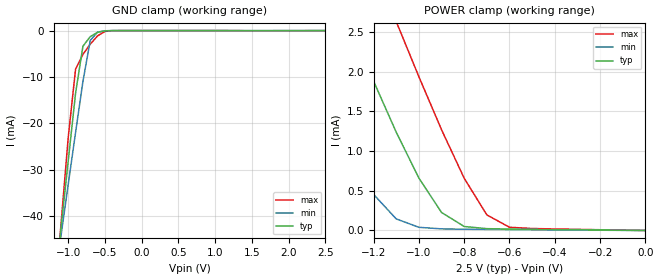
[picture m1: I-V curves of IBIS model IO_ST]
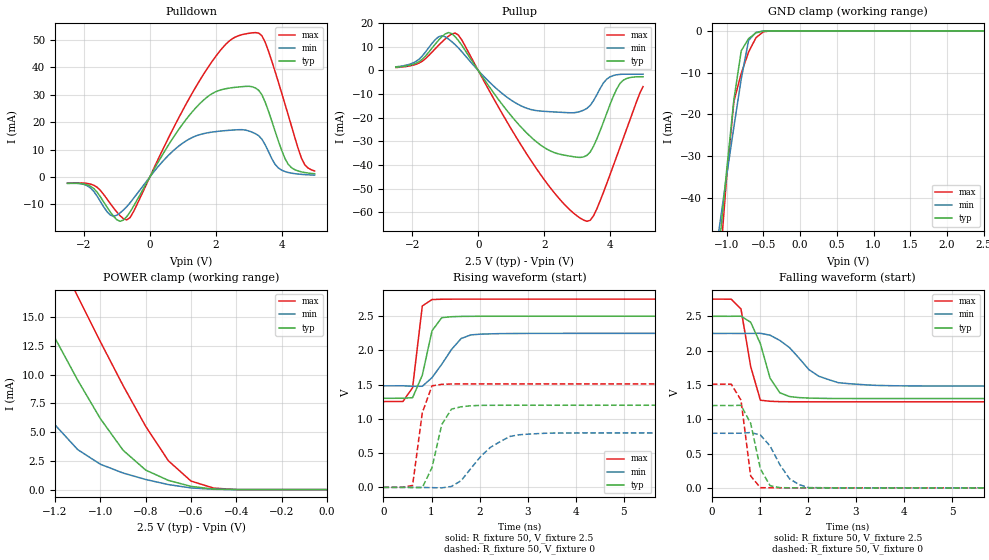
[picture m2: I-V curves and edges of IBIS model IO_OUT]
[IBIS Ver]   3.2
[Comment Char]   |_char
[File name]   sg5032can25.ibs
[File Rev]   1.0
[Date]   2015/11/24 22:00:00
[Source]
[Notes]
[Disclaimer]
This information is for modeling purposes only, and is not guaranteed.
Property of SEIKO EPSON Corp.,
unauthorized reproduction and/or distribution is strictly prohibited.
[Copyright]
Copyright 2006, SEIKO EPSON Corp.
[Component]   SG5032CAN
Si_location Pin
Timing_location Pin
[Manufacturer]   SEIKO EPSON Corp.
| COG
| COG
[Package]
R_pkg   56.75m   56.75m   56.75m
L_pkg   2.25n   2.25n   2.25n
C_pkg   0.860p   0.860p   0.860p
[Pin] signal_name   model_name
1   /ST   IO_ST
2   GND   GND
3   OUT   IO_OUT
4   Vcc   POWER
| Models and submodels in the file (2): IO_ST (Input), IO_OUT (3-state)
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[Model]   IO_ST
Model_type Input
Polarity Inverting
Vinh=2.00
Vinl=0.50
C_comp   5p   4p   6p
[Temperature Range] 25   105   -40
[Voltage Range]   2.5   2.25   2.75
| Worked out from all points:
|   GND clamp passes 1 mA (typ) near -0.67 V on its own axis
|   POWER clamp passes 1 mA (typ) near -1.06 V on its own axis
[GND Clamp]
-2.5V     -258mA     -212mA     -315.4mA
-1.2V     -57.55mA   -55.73mA   -61.1mA
-1.1V     -42.76mA   -44.37mA   -42.03mA
-1V       -28.06mA   -33.1mA    -23.01mA
-900mV    -13.48mA   -21.96mA   -8.306mA
-800mV    -3.366mA   -10.96mA   -5.116mA
-700mV    -1.291mA   -2.106mA   -2.915mA
-600mV    -372.4uA   -316.5uA   -1.133mA
-500mV    -49.9uA    -42.12uA   -183.6uA
-400mV    -3.838uA   -5.008uA   -10.26uA
2.5V      36.41pA    4.239uA    -10.27uA
[POWER Clamp]
-2.5V     10.82mA    8.867mA    12.49mA
-1.6V     4.625mA    2.831mA    6.156mA
-1.5V     3.936mA    2.166mA    5.451mA
-1.3V     2.559mA    943.7uA    4.043mA
-1.2V     1.882mA    455uA      3.338mA
-1.1V     1.239mA    146uA      2.634mA
-1V       661uA      40.15uA    1.938mA
-900mV    227.3uA    20.05uA    1.27mA
-800mV    50.18uA    15.52uA    658.6uA
-700mV    22.76uA    13.11uA    196.3uA
-600mV    17.66uA    11.02uA    40.37uA
0V        36.41pA    613.4pA    26.22pA
[Model]   IO_OUT
Model_type 3-state
Enable Active-High
Polarity Non-Inverting
Vmeas=1.25
C_comp   5p   4p   6p
[Temperature Range] 25   105   -40
[Voltage Range]   2.5   2.25   2.75
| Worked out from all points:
|   slope of the pulldown table from 0 to 0.375 V, typ, clamps not added: 47.4 ohm
|   slope of the pullup table from 0 to 0.375 V, typ, clamps not added: 48.9 ohm
|   GND clamp passes 1 mA (typ) near -0.64 V on its own axis
|   POWER clamp passes 1 mA (typ) near -0.72 V on its own axis
|   falling waveform, R_fixture 50, V_fixture 2.5: 20-80 % time 358ps typ, 689ps min, 253ps max; typ from 2.5 V to 1.3 V
|   falling waveform, R_fixture 50, V_fixture 0: 20-80 % time 246ps typ, 411ps min, 166ps max; typ from 1.2 V to 0 V
|   rising waveform, R_fixture 50, V_fixture 2.5: 20-80 % time 253ps typ, 473ps min, 152ps max; typ from 1.3 V to 2.5 V
|   rising waveform, R_fixture 50, V_fixture 0: 20-80 % time 274ps typ, 666ps min, 211ps max; typ from 0 V to 1.2 V
[Pullup]
-2.5V     1.374mA    1.541mA    1.237mA
-1.8V     3.697mA    4.727mA    3.1mA
-1.1V     14.34mA    14.7mA     12.08mA
-600mV    12.65mA    9.537mA    14.98mA
600mV     -12.02mA   -8.251mA   -15.16mA
1.6V      -28.19mA   -16.55mA   -38.12mA
2.4V      -35.2mA    -17.64mA   -53.34mA
3.3V      -35.93mA   -16.04mA   -63.89mA
3.6V      -28.95mA   -10.25mA   -58.57mA
3.9V      -18.1mA    -3.658mA   -47.9mA
4.3V      -5.531mA   -1.653mA   -32.62mA
5V        -2.656mA   -1.579mA   -6.836mA
[Pulldown]
-2.5V     -2.36mA    -2.211mA   -2.183mA
-1.7V     -4.229mA   -5.289mA   -3.031mA
-1.1V     -14.37mA   -14.35mA   -11.31mA
-600mV    -12.8mA    -9.427mA   -14.81mA
600mV     12.32mA    8.312mA    15.08mA
1.5V      26.57mA    15.39mA    34.96mA
2.4V      32.41mA    17.02mA    49.52mA
3.2V      32.49mA    15.82mA    52.7mA
3.5V      27.3mA     11.76mA    49.18mA
4.2V      4.583mA    1.63mA     22.55mA
4.6V      1.865mA    952uA      6.872mA
5V        1.18mA     668.2uA    2.194mA
[GND Clamp]
-2.5V     -322.6mA   -266mA     -388.9mA
-1.1V     -51.71mA   -47.32mA   -58.37mA
-1V       -33.72mA   -34.9mA    -35.42mA
-900mV    -16.51mA   -23.04mA   -16.92mA
-800mV    -4.792mA   -11.52mA   -10.2mA
-700mV    -1.863mA   -2.312mA   -5.089mA
-600mV    -506.1uA   -360.8uA   -1.661mA
-500mV    -63.67uA   -48.09uA   -236uA
-400mV    -4.383uA   -5.495uA   -11.57uA
2.5V      129.9pA    52.78nA    86.58pA
[POWER Clamp]
-2.5V     66.42mA    55.67mA    75.3mA
-1.6V     28.98mA    19.26mA    37.34mA
-1.5V     24.93mA    15.49mA    33.18mA
-1.3V     17.01mA    8.534mA    24.92mA
-1.2V     13.18mA    5.632mA    20.85mA
-1.1V     9.527mA    3.483mA    16.82mA
-900mV    3.431mA    1.446mA    9.067mA
-800mV    1.7mA      880.4uA    5.505mA
-700mV    803.8uA    438uA      2.511mA
-600mV    280.8uA    145.5uA    743uA
-500mV    45.47uA    25.7uA     130.4uA
0V        129.9pA    720.2pA    126pA
[Falling Waveform]
R_fixture=50
V_fixture=2.5
V_fixture_min=2.25
V_fixture_max=2.75
0s        2.5V       2.25V      2.75V
404ps     2.5V       2.25V      2.749V
606.1ps   2.502V     2.249V     2.607V
808.1ps   2.413V     2.251V     1.768V
1.01ns    2.1V       2.252V     1.277V
1.212ns   1.596V     2.225V     1.262V
1.414ns   1.386V     2.148V     1.256V
2.222ns   1.305V     1.628V     1.254V
3.232ns   1.301V     1.5V       1.254V
20ns      1.301V     1.483V     1.254V
[Falling Waveform]
R_fixture=50
V_fixture=0
V_fixture_min=0
V_fixture_max=0
0s        1.2V       795.4mV    1.511V
404ps     1.199V     794.9mV    1.511V
606.1ps   1.203V     796.4mV    1.279V
808.1ps   941.2mV    806.2mV    172.9mV
1.01ns    276mV      770.6mV    2.78mV
1.212ns   31.84mV    609.3mV    782.8uV
1.414ns   3.046mV    338.7mV    222.8uV
1.616ns   1.153mV    132.1mV    -8.828uV
2.02ns    269.5uV    4.004mV    7.436uV
20ns      -1.408uV   -37.66uV   11.39uV
[Rising Waveform]
R_fixture=50
V_fixture=2.5
V_fixture_min=2.25
V_fixture_max=2.75
0s        1.301V     1.483V     1.254V
404ps     1.302V     1.484V     1.254V
606.1ps   1.311V     1.477V     1.457V
808.1ps   1.638V     1.477V     2.65V
1.01ns    2.287V     1.603V     2.744V
1.212ns   2.479V     1.798V     2.749V
1.414ns   2.493V     2.013V     2.75V
1.616ns   2.497V     2.175V     2.75V
2.02ns    2.5V       2.238V     2.75V
20ns      2.5V       2.25V      2.75V
[Rising Waveform]
R_fixture=50
V_fixture=0
V_fixture_min=0
V_fixture_max=0
0s        0V         0V         0V
606.1ps   -3.406mV   956.5uV    28.2mV
808.1ps   -3.534mV   -1.102mV   1.091V
1.01ns    288.9mV    -4.386mV   1.483V
1.212ns   916.8mV    -7.249mV   1.505V
1.414ns   1.143V     13.49mV    1.51V
1.616ns   1.177V     98.01mV    1.511V
2.222ns   1.199V     583.8mV    1.511V
3.03ns    1.2V       778.2mV    1.511V
20ns      1.2V       795.4mV    1.511V
[Ramp]
R_load=50
dV/dt_r   7.198E-1/2.473E-10   4.773E-1/6.620E-10   9.067E-1/1.507E-10
dV/dt_f   7.191E-1/3.226E-10   4.600E-1/6.603E-10   8.976E-1/1.949E-10
|[End   IO_OUT
